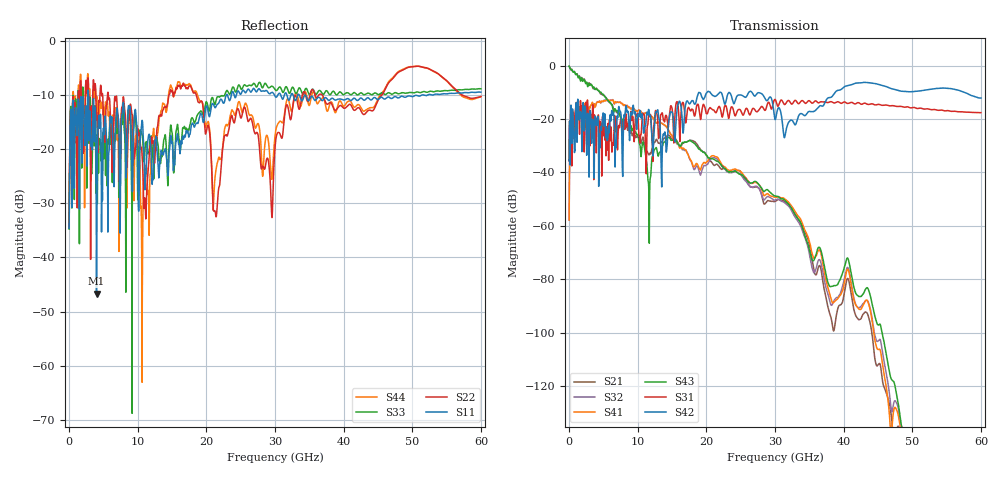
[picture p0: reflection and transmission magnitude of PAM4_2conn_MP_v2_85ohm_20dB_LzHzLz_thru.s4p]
! Info: Touchstone file created by Circ.  Input file=FAB50GbE_2conn_Midplane_Examax_Topo2_v2_85ohm_20dB_LzHzLz.circ
# Hz S RI R 50
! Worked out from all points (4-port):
!   6000 points, 10 MHz to 60 GHz, reference 50 ohm
!   strongest paths, dB at 10 MHz, 15.01 GHz, 30.01 GHz, 45.01 GHz, 60 GHz:
!     S42: -35.6, -17.4, -20.2, -7.0, -12.1
!     S31: -35.7, -16.0, -12.6, -14.5, -17.6
!     S43: -0.2, -27.9, -48.8, -97.1, -156.3
!     S41: -57.8, -26.4, -49.2, -106.3, -159.7
!     S32: -57.8, -26.4, -50.3, -103.2, -150.5
!     S21: -0.2, -27.4, -50.8, -112.1, -148.7
!   lowest |S11| = -46.7 dB at 4 GHz (marker M1), VSWR 1.01, Z = 49.9 - j0.45 ohm
!   |S11| at or under -10 dB: start of sweep to 2.736 GHz; 2.823 GHz to 22.9 GHz (20.08 GHz wide, 156 % of centre); 34.43 GHz to 51.37 GHz (16.94 GHz wide, 39.5 % of centre)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
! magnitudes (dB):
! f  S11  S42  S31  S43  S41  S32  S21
! 10 MHz  -34.6  -35.6  -35.7  -0.2  -57.8  -57.8  -0.2
! 4 GHz  -46.7  -22.4  -27.3  -8.8  -14.0  -13.9  -8.5
! 10.65 GHz  -14.7  -18.2  -19.0  -29.9  -18.3  -18.2  -27.4
! 14.8 GHz  -17.5  -17.3  -15.1  -27.8  -25.7  -25.8  -26.9
! 21.29 GHz  -12.3  -11.5  -17.4  -35.4  -34.1  -34.7  -37.2
! 37.2 GHz  -10.6  -14.3  -13.6  -75.1  -77.5  -80.4  -84.1
! 60 GHz  -9.5  -12.1  -17.6  -156.3  -159.7  -150.5  -148.7
